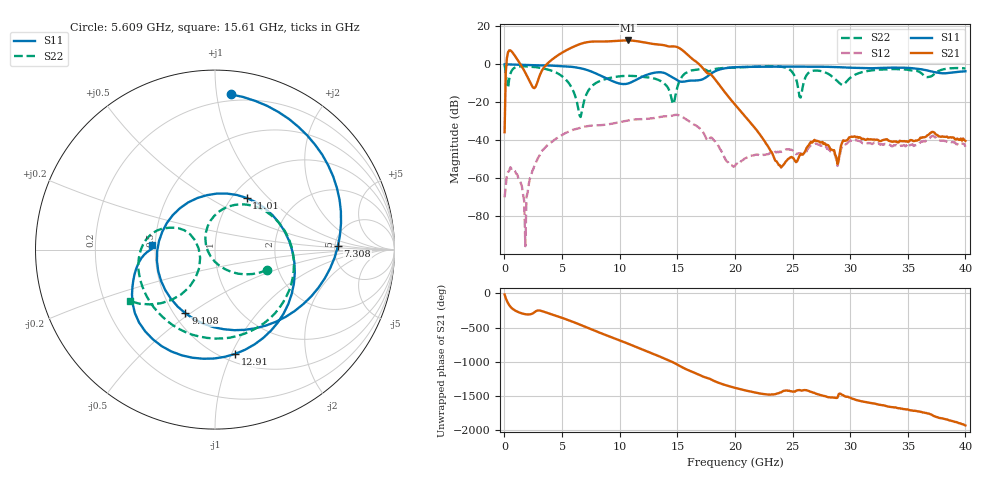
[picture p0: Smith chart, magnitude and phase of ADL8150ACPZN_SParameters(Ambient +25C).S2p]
! Analog Devices, Inc.
! Device:	ADL8150ACPZN
! Description:	"GaAs, HBT, MMIC, Low Phase Noise Amplifier, 6 GHz to 14 GHz"
! Conditions:	Vcc = 5.0 V
!		Icc = 74 mA quiescent (Self-biased mode)
!		Pin = -20 dBm
!		Operating Temperature = +25 C (at package bottom)
! Product validation unit SN19 soldered down to Evaluation Board as shown on ADL8150-EVALZ User Guide. Board loss de-embedded from S21 magnitude.  All other RF measurements reference to RF coaxial connector.
! Frequency (GHz)	S11_Mag (dB)	S11_Phase (deg)	S21_Mag (dB)	S21_Phase (deg)	S12_Mag (dB)	S12_Phase (deg)	S22_Mag (dB)	S22_Phase (deg)
#  GHZ  S  DB  R 50
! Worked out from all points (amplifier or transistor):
!   401 points, 10 MHz to 40 GHz, reference 50 ohm
!   highest |S21| = 12.5 dB at 10.71 GHz (marker M1)
!   |S21| within 3 dB of that: 6.104 GHz to 14.15 GHz (8.049 GHz wide, 79.5 % of centre)
!   unconditionally stable (mu >= 1): start of sweep to end of sweep
!   at 6.608 GHz: K = 2.63, MAG = 15.0 dB, |S12| = -33.4 dB
!   at 20 GHz: K = 266.05, MAG = -11.1 dB, |S12| = -53.5 dB
!   at 40 GHz: K = 1699.40, MAG = -33.8 dB, |S12| = -43.4 dB
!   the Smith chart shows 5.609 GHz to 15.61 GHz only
!   S11 on the Smith chart (normalised r, x): 5.609 GHz: 0.15, +1.09; 7.308 GHz: 5.32, +0.36; 9.108 GHz: 0.57, -0.48; 11.01 GHz: 1.16, +0.76; 12.91 GHz: 0.58, -1.03; 15.61 GHz: 0.48, +0.03
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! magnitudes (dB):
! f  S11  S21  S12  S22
! 10 MHz  0.0  -35.7  -70.0  -0.2
! 309.9 MHz  -0.1  6.4  -56.7  -12.4
! 509.9 MHz  -0.1  7.3  -54.1  -5.0
! 1.81 GHz  -0.3  -4.4  -95.7  -1.1
! 3.109 GHz  -0.6  -5.1  -47.3  -1.9
! 5.609 GHz  -1.2  8.1  -35.3  -10.1
! 6.708 GHz  -2.2  11.0  -33.1  -24.8
! 7.308 GHz  -3.3  11.8  -32.4  -13.5
! 9.108 GHz  -8.1  12.1  -31.5  -7.2
! 10.71 GHz  -10.1  12.5  -29.6  -6.1
! 11.01 GHz  -9.4  12.5  -29.3  -6.1
! 12.91 GHz  -4.6  10.7  -28.3  -7.4
! 13.41 GHz  -4.2  10.4  -27.8  -8.4
! 14.61 GHz  -6.9  9.4  -26.9  -20.8
! 15.61 GHz  -9.1  6.6  -28.3  -5.1
! 20.1 GHz  -1.5  -21.9  -52.3  -1.7
! 23.9 GHz  -1.2  -53.1  -45.8  -1.2
! 25.7 GHz  -1.2  -47.2  -46.9  -17.5
! 26.7 GHz  -1.3  -41.2  -42.4  -3.5
! 28.9 GHz  -1.5  -52.5  -53.5  -9.0
! 33.4 GHz  -1.8  -40.3  -42.3  -2.6
! 40 GHz  -3.7  -40.3  -43.4  -2.2
